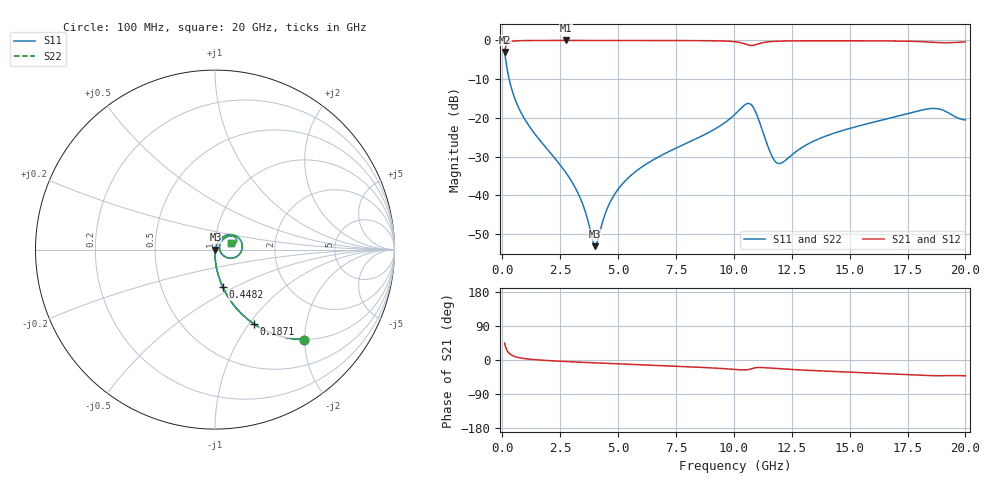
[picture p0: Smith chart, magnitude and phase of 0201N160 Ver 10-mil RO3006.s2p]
# GHz S MA R 50
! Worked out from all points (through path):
!   1601 points, 100 MHz to 20 GHz, reference 50 ohm
!   highest |S21| = -0.02 dB at 2.737 GHz (marker M1); lowest = -3.0 dB at 100 MHz (marker M2)
!   group delay of S21, straight-line fit = 6.77 ps
!   lowest |S11| = -53.1 dB at 4.018 GHz (marker M3), VSWR 1.00, Z = 50.2 - j0.0273 ohm
!   |S11| at or under -10 dB: 296 MHz to end of sweep
!   |S22| runs from -53.1 to -3.0 dB; largest |S21 - S12| = 0
!   S11 on the Smith chart (normalised r, x): 100 MHz: 1.00, -1.98; 187.1 MHz: 1.00, -1.06; 448.2 MHz: 1.00, -0.44; 20 GHz: 1.19, +0.09
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0.1  0.7039 -45.4  0.7097 44.6  0.7097 44.6  0.7039 -45.4
0.1870625  0.4676 -62.4  0.8832 27.5  0.8832 27.5  0.4676 -62.4
0.2865625  0.3256 -71.4  0.9448 18.5  0.9448 18.5  0.3256 -71.4
0.44825  0.2135 -78.3  0.9761 11.5  0.9761 11.5  0.2135 -78.3
1.107438  0.08271 -86.6  0.9954 2.6  0.9954 2.6  0.08271 -86.6
2.73675  0.01987 -88.9  0.9979 -4.0  0.9979 -4.0  0.01987 -88.9
3.420812  0.008459 -82.2  0.9979 -6.0  0.9979 -6.0  0.008459 -82.2
3.918312  0.002528 -37.5  0.9977 -7.3  0.9977 -7.3  0.002528 -37.5
4.017812  0.002218 -7.0  0.9977 -7.6  0.9977 -7.6  0.002218 -7.0
4.52775  0.006732 60.3  0.9975 -8.9  0.9975 -8.9  0.006732 60.3
4.9755  0.01174 67.5  0.9973 -10.0  0.9973 -10.0  0.01174 67.5
5.696875  0.01968 69.9  0.9969 -11.9  0.9969 -11.9  0.01968 69.9
6.741625  0.03137 69.4  0.996 -14.5  0.996 -14.5  0.03137 69.4
10.05  0.1115 47.9  0.9612 -25.0  0.9612 -25.0  0.1115 47.9
10.53506  0.1511 20.6  0.8899 -26.1  0.8899 -26.1  0.1511 20.6
10.78381  0.1447 -5.9  0.8603 -22.6  0.8603 -22.6  0.1447 -5.9
11.60469  0.03409 -24.1  0.9656 -21.6  0.9656 -21.6  0.03409 -24.1
11.90319  0.02591 3.5  0.9764 -22.9  0.9764 -22.9  0.02591 3.5
13.37081  0.04896 50.6  0.9886 -27.7  0.9886 -27.7  0.04896 50.6
16.69162  0.09879 46.8  0.9834 -36.6  0.9834 -36.6  0.09879 46.8
18.65675  0.1325 27.2  0.944 -41.6  0.944 -41.6  0.1325 27.2
20  0.09425 23.4  0.9562 -41.7  0.9562 -41.7  0.09425 23.4
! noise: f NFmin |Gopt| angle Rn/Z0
0.1  0.0005667  0.9246  0.3639  0.001666
2.301  0.003834  0.7648  4.412  0.003307
4.515  0.006521  0.7339  8.507  0.004865
6.729  0.009402  0.7268  12.59  0.006762
8.943  0.01639  0.7855  16.7  0.01538
11.14  0.06079  0.9228  20.88  0.1686
13.36  0.02275  0.7733  24.85  0.01956
15.57  0.02307  0.7453  28.75  0.0171
17.79  0.03829  0.8188  32.78  0.04075
20  0.05555  0.8577  36.78  0.0752
